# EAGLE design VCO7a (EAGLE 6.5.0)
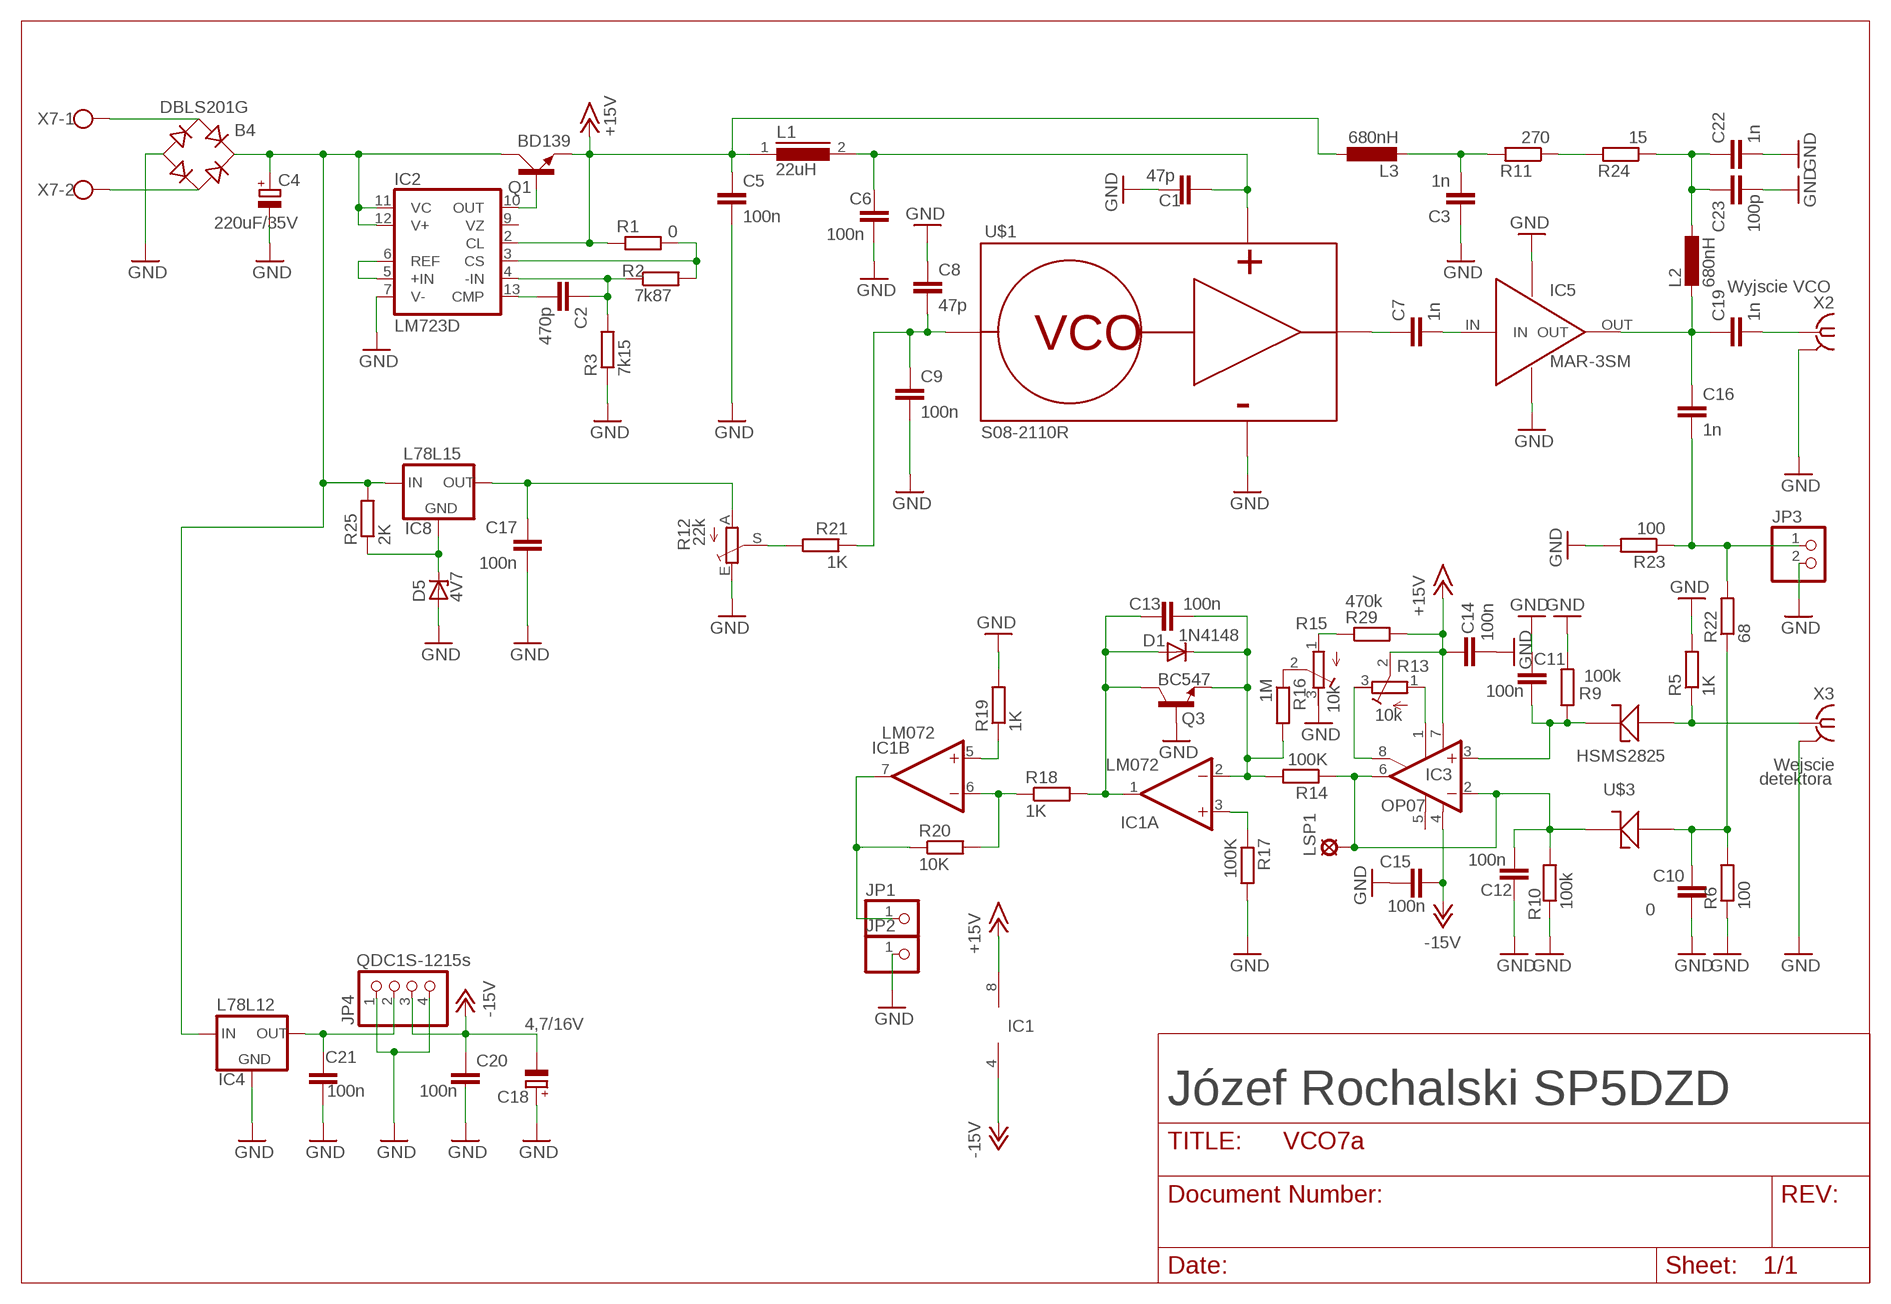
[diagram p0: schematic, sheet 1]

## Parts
B4  DBLS201G  [DBS]
C1  47p  C-EUC1812  [C1812]
C2  470p  C-EUC1206K  [C1206K]
C3  1n  C-EUC1206K  [C1206K]
C4  220uF/35V  CPOL-EU140CLH-1010  [140CLH-1010]
C5  100n  C-EUC1206K  [C1206K]
C6  100n  C-EUC1206K  [C1206K]
C7  1n  C-EUC1206K  [C1206K]
C8  47p  C-EUC1812  [C1812]
C9  100n  C-EUC1206K  [C1206K]
C10  0  C-EUC1206K  [C1206K]
C11  100n  C-EUC1206K  [C1206K]
C12  100n  C-EUC1206K  [C1206K]
C13  100n  C-EUC1206K  [C1206K]
C14  100n  C-EUC1206K  [C1206K]
C15  100n  C-EUC1206K  [C1206K]
C16  1n  C-EUC1206K  [C1206K]
C17  100n  C-EUC1206K  [C1206K]
C18  4,7/16V  CPOL-EUCT6032  [CT6032]
C19  1n  C-EUC1206  [C1206]
C20  100n  C-EUC1206K  [C1206K]
C21  100n  C-EUC1206K  [C1206K]
C22  1n  C-EUC1206K  [C1206K]
C23  100p  C-EUC1206K  [C1206K]
D1  1N4148  DIODE-MELF-MLL41  [MELF-MLL41]
D5  4V7  1N4728  [DO41Z10]
IC1  LM072  TL072D  [SO08]
IC2  LM723D  [SO14]
IC3  OP07  OP07CR  [SO08]
IC4  L78L12  L78LXXCZ/BZ  [TO92]
IC5  MAR-3SM  MMIC  [MMIC]
IC8  L78L15  L78LXXCZ/BZ  [TO92]
JP1  PINHD-1X01_2.54  [1X01]
JP2  PINHD-1X01_2.54  [1X01]
JP3  PINHD-1X2  [1X02]
JP4  QDC1S-1215s  PINHD-1X4  [1X04]
L1  22uH  EMC9714  [EMC9714]
L2  680nH  L-EUL4035M  [L4035M]
L3  680nH  L-EUL4035M  [L4035M]
LSP1  SE11  [SE11]
Q1  BD139  [TO126AV]
Q3  BC547  BC847CSMD  [SOT23]
R1  0  R-EU_R1206  [R1206]
R2  7k87  R-EU_R1206  [R1206]
R3  7k15  R-EU_R1206  [R1206]
R5  1K  R-EU_R1206  [R1206]
R6  100  R-EU_R1206  [R1206]
R9  100k  R-EU_R1206  [R1206]
R10  100k  R-EU_R1206  [R1206]
R11  270  R-EU_R1206  [R1206]
R12  22k  TRIM_EU-PT10S  [PT-10S]
R13  10k  R-TRIMM64W  [RTRIM64W]
R14  100K  R-EU_R1206  [R1206]
R15  10k  R-TRIMM64W  [RTRIM64W]
R16  1M  R-EU_R1206  [R1206]
R17  100K  R-EU_R1206  [R1206]
R18  1K  R-EU_R1206  [R1206]
R19  1K  R-EU_R1206  [R1206]
R20  10K  R-EU_R1206  [R1206]
R21  1K  R-EU_R1206  [R1206]
R22  68  R-EU_R1206  [R1206]
R23  100  R-EU_R1206  [R1206]
R24  15  R-EU_R1206  [R1206]
R25  2K  R-EU_R1206  [R1206]
R29  470k  R-EU_R1206  [R1206]
U$1  S08-2110R  [S08-2110R]
U$3  HSMS2825  [HSMS2825]
X2  SMA-142-0701-801/806  [J502-ND-142-0701-801/806]
X3  BNC  SMA-142-0701-801/806  [J502-ND-142-0701-801/806]
X7  AK300/2  [AK300/2]

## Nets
+15V: C5.1 C14.1 IC1.8(P:V+) IC2.2(CL) IC3.7(V+) L1.1 L3.1 Q1.E R1.1 R13.2(S) R29.2
-12V: C15.2 C18.- C20.1 IC1.4(P:V-) IC3.4(V-) JP4.3 ; supply symbol labelled -15V
GND: B4.- C1.2 C3.1 C4.- C5.2 C6.2 C8.1 C9.2 C10.2 C11.1 C12.2 C14.2 C15.1 C17.2 C18.+ C20.2 C21.2 C22.2 C23.2 D5.A IC2.7(V-) IC4.2(GND) IC5.GND IC5.GND1 JP2.1 JP3.2 JP4.1 JP4.4 Q3.1(B) R3.1 R5.2 R6.1 R9.2 R10.1 R12.E R15.3(E) R17.2 R19.2 R23.2 U$1.P$4(GND) X2.G@1 X2.G@2 X2.G@3 X2.G@4 X3.G@1 X3.G@2 X3.G@3 X3.G@4
N$1: IC2.5(+IN) IC2.6(REF)
N$2: IC2.10(OUT) Q1.B
N$3: R12.S R21.2
N$4: C7.1 U$1.P$3(OUT)
N$5: C2.2 IC2.13(CMP)
N$6: C2.1 IC2.4(-IN) R2.1 R3.2
N$7: IC2.3(CS) R1.2 R2.2
N$8: C16.2 JP3.1 R22.2 R23.1
N$10: C3.2 L3.2 R11.2
N$11: C17.1 IC8.1(OUT) R12.A
N$12: D5.C IC8.2(GND) R25.1
N$13: C1.1 C6.1 L1.2 U$1.P$2(VCC)
N$14: R5.1 U$3.P$4(A2) X3.1
N$15: B4.+ C4.+ IC2.11(VC) IC2.12(V+) IC4.3(IN) IC8.3(IN) Q1.C R25.2
N$17: C8.2 C9.1 R21.1 U$1.P$1(CONTROL)
N$18: C10.1 R6.2 R22.1 U$3.P$3(A1)
N$19: IC3.8(ON2) R13.3(E)
N$20: C12.1 IC3.2(-IN) IC3.6(OUT) LSP1.MP R10.2 R14.1 U$3.P$2(K1)
N$21: C13.2 D1.C IC1.2(A:-IN) Q3.2(E) R14.2 R16.2
N$22: R15.2(S) R16.1
N$23: C16.1 C19.1 IC5.OUT L2.2
N$26: IC1.3(A:+IN) R17.1
N$27: C13.1 D1.A IC1.1(A:OUT) Q3.3(C) R18.2
N$28: R11.1 R24.2
N$29: IC1.6(B:-IN) R18.1 R20.2
N$30: IC1.5(B:+IN) R19.1
N$31: IC1.7(B:OUT) JP1.1 R20.1
N$32: IC3.1(ON1) R13.1(A)
N$33: R15.1(A) R29.1
N$34: C19.2 X2.1
N$35: C22.1 C23.1 L2.1 R24.1
N$36: C21.1 IC4.1(OUT) JP4.2
N$37: C11.2 IC3.3(+IN) R9.1 U$3.P$1(K2)
N$41: C7.2 IC5.IN
N$44: B4.AC1 X7.1
N$45: B4.AC2 X7.2
Unconnected: IC2.9(VZ) IC3.5(OPT)

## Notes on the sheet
- Wyjscie VCO
- Wejscie
- detektora
- IC1
- Józef Rochalski SP5DZD

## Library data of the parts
B4 = rectifier:DB?*G: Single Phase 1.0 AMP Glass Passivated Bridge Rectifier Taiwan Semiconductor Co.,Ltd. - TSC Source: http://www.taiwansemi.com/TSCbig5/ezcatfiles/cust/img/img/db101g.pdf http://www.ts.com.tw/db/pictures/modules/PDT/PDT060207001/DBLS201G.pdf
C1-C3 C5-C17 C19-C23 = rcl:C-EU: CAPACITOR, European symbol
C4 C18 = rcl:CPOL-EU: POLARIZED CAPACITOR, European symbol
D1 = diode-1:DIODE-: DIODE
D5 = diode-1:1N4728: Z DIODE
IC1 = linear:TL072: OP AMP
IC2 = linear:*723: Positive VOLTAGE REGULATOR
IC3 = linear3:OP07*: OP AMP
IC4 IC8 = v-reg-3:L78LXXCZ/BZ: VOLTAGE REGULATOR
IC5 = MMIC1:MMIC
JP1 JP2 = pinhead-2:PINHD-1X01: PIN HEADER
JP3 = pinhead:PINHD-1X2: PIN HEADER
JP4 = pinhead:PINHD-1X4: PIN HEADER
L1 = inductors:EMC9714: INDUCTOR
L2 L3 = rcl:L-EU: INDUCTOR, European symbol
LSP1 = solpad:SE11: SOLDER PAD
Q1 = transistor-power:BD139: NPN TRANSISTOR
Q3 = transistor-npn:BC847*: NPN Transistor
R1-R3 R5 R6 R9-R11 R14 R16-R25 R29 = rcl:R-EU_: RESISTOR, European symbol
R12 = pot:TRIM_EU-: POTENTIOMETER
R13 R15 = rcl:R-TRIMM: Trimm resistor
U$1 = S08-2110R:S08-2110R: VCO AGILENT S08-2110R 0.8-1.2GHz
U$3 = HSMS2825:HSMS2825
X2 X3 = con-coax:SMA-: SMA 50 Ohm End Launch Jack Receptacle - Round Contact; MF: JOHNSON COMPONENTS; MPN: 142-0701-801; OC_FARNELL: 1608592; OC_NEWARK: 90F2624
X7 = con-ptr500+:AK300/2: CONNECTOR

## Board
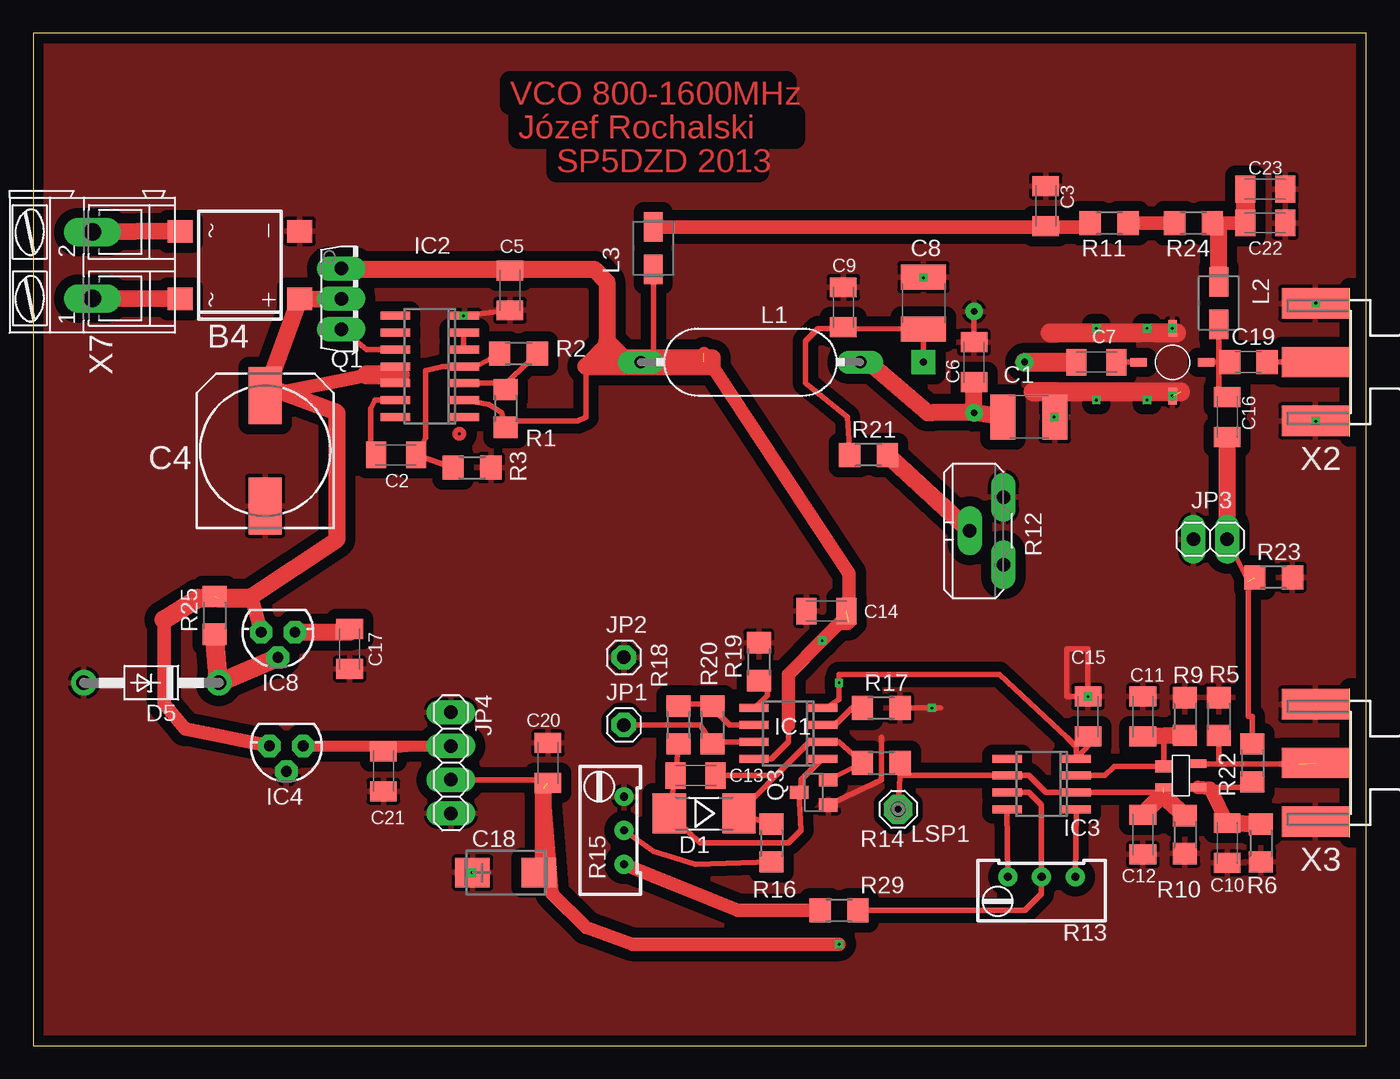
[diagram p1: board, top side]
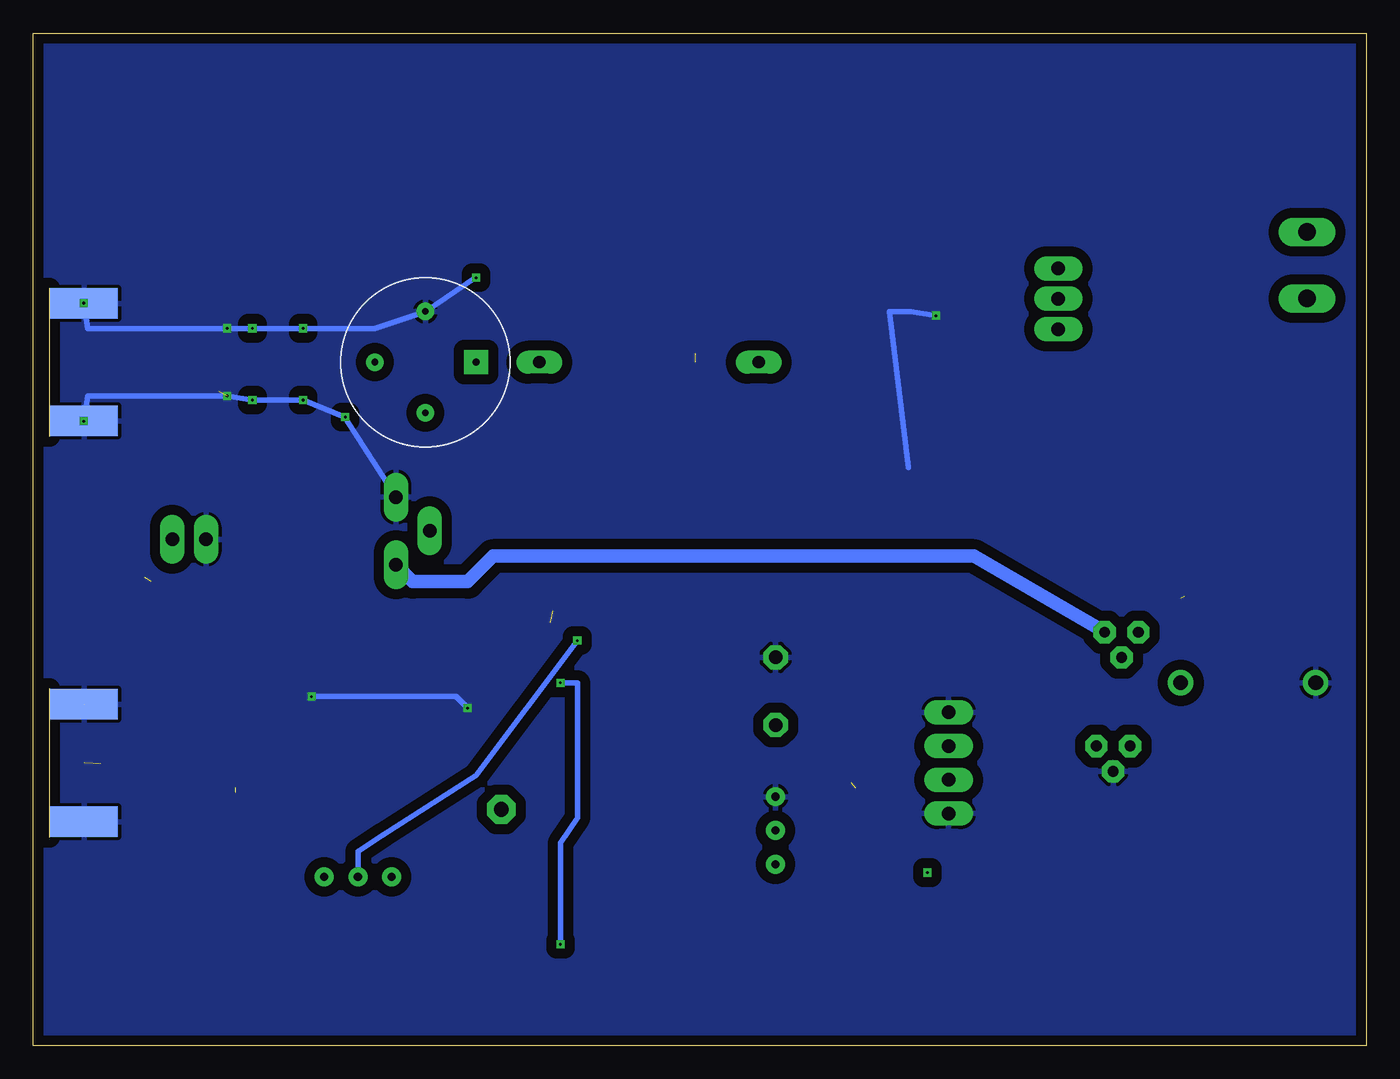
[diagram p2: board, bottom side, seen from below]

Size 100.32 x 76.19 mm. Coordinates in mm from the lower left corner, seen from the top.
Outline: 0,0 100.32,0 100.32,76.19 0,76.19 0,0
Copper layers (1*16): Top 0.035mm / dielectric 1.5mm / Bottom 0.035mm
Design rules "default *": minimum track width 16mil, minimum drill 8mil, track to track 16mil, track to pad 8mil, pad to pad 8mil, via to via 8mil, smd to smd 8mil, copper to edge 10mil, drill to drill 8mil, minimum pad ring 16mil, minimum via ring 8mil, stop-mask expansion 4mil, vias tented up to drill 0mil, thermal gap 10mil

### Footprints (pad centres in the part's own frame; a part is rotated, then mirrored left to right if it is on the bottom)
DBS = smd 1.7 x 1.9: + -2.55,-4.5; - 2.55,-4.5; AC1 -2.55,4.5; AC2 2.55,4.5
C1812 = smd 1.9 x 3.4: 1 -1.95,0; 2 1.95,0
C1206K = smd 1.5 x 2: 1 -1.5,0; 2 1.5,0
140CLH-1010 = smd 4.3 x 2.5: + 4.15,0; - -4.15,0
CT6032 = smd 2.6 x 2.2: + -2.5,0; - 2.5,0
C1206 = smd 1.6 x 1.8: 1 -1.4,0; 2 1.4,0
MELF-MLL41 = smd 2.5 x 3: A 2.625,0; C -2.625,0
DO41Z10 = drill 1.118: A 5.08,0; C -5.08,0
SO08 = smd 0.6 x 2.2: 1 -1.905,-2.6; 2 -0.635,-2.6; 3 0.635,-2.6; 4 1.905,-2.6; 5 1.905,2.6; 6 0.635,2.6; 7 -0.635,2.6; 8 -1.905,2.6
SO14 = smd 0.6 x 2.2: 1 -3.81,-2.6; 2 -2.54,-2.6; 3 -1.27,-2.6; 4 0,-2.6; 5 1.27,-2.6; 6 2.54,-2.6; 7 3.81,-2.6; 8 3.81,2.6; 9 2.54,2.6; 10 1.27,2.6; 11 0,2.6; 12 -1.27,2.6; 13 -2.54,2.6; 14 -3.81,2.6
TO92 = drill 0.813 pad 1.676 octagon: 1 -1.27,0; 2 0,1.905; 3 1.27,0
MMIC = smd 0.635 x 1.27: GND 0,2.54; GND1 0,-2.54 | smd 1.27 x 0.635: IN -2.54,0; OUT 2.54,0
1X01 = drill 1.016 octagon: 1 0,0
1X02 = drill 1.016 long: 1 -1.27,0; 2 1.27,0
1X04 = drill 1.016 long: 1 -3.81,0; 2 -1.27,0; 3 1.27,0; 4 3.81,0
EMC9714 = drill 0.914 long: 1 -8.255,0; 2 8.255,0
L4035M = smd 2.2 x 1.4: 1 -1.6,0; 2 1.6,0
SE11 = drill 1.118 pad 2.159 octagon: MP 0,0
TO126AV = drill 1.016 long: B 2.286,-1.27; C 0,-1.27; E -2.286,-1.27
SOT23 = smd 1 x 1.4: 1 -0.95,-1.1; 2 0.95,-1.1; 3 0,1.1
R1206 = smd 1.6 x 1.803: 1 -1.422,0; 2 1.422,0
PT-10S = drill 1.016 long: A -2.54,-1.27; E 2.54,-1.27; S 0,1.27
RTRIM64W = drill 0.61: 1 1.27,-2.54; 2 1.27,0; 3 1.27,2.54
S08-2110R = drill 0.5 pad 1.778 square: P$1 -3.81,0 | drill 0.5 pad 1.27: P$2 0,3.81; P$3 3.81,0; P$4 0,-3.81
HSMS2825 = smd 0.914 x 1.27: P$1 -0.699,-1.27 | smd 0.635 x 1.27: P$2 0.889,-1.27; P$3 0.889,1.27; P$4 -0.889,1.27
J502-ND-142-0701-801/806 = smd 5.08 x 2.286: 1 2.565,0; G@1 2.565,4.42; G@2 2.565,-4.42 | smd 5.08 x 2.286 bottom: G@3 2.565,4.42; G@4 2.565,-4.42
AK300/2 = drill 1.321 long: 1 -2.515,0; 2 2.489,0

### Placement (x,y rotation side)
B4  15.56,58.74 90 top
C1  74.93,47.31 0 top
C2  27.3,44.45 180 top
C3  76.2,63.18 270 top
C4  17.46,44.77 90 top
C5  35.88,56.83 270 top
C6  70.8,51.44 90 top
C7  80.01,51.44 0 top
C8  66.99,55.88 270 top
C9  60.96,55.56 90 top
C10  89.85,15.24 270 top
C11  83.5,24.77 270 top
C12  83.5,15.88 270 top
C13  49.85,20.32 0 top
C14  59.69,32.7 180 top
C15  79.38,24.77 270 top
C16  89.85,47.31 270 top
C17  23.81,29.84 270 top
C18  35.56,13.02 0 top
C19  91.44,51.44 0 top
C20  38.73,21.27 90 top
C21  26.35,20.64 270 top
C22  92.71,61.91 0 top
C23  92.71,64.45 0 top
D1  50.48,17.46 180 top
D5  8.89,27.3 180 top
IC1  56.83,23.5 90 top
IC2  29.84,51.12 90 top
IC3  75.88,19.68 90 top
IC4  19.05,22.54 180 top
IC5  85.72,51.44 0 top
IC8  18.41,31.11 180 top
JP1  44.45,24.13 0 top
JP2  44.45,29.21 0 top
JP3  88.58,38.1 180 top
JP4  31.43,21.27 270 top
L1  53.98,51.44 0 top
L2  89.22,55.88 270 top
L3  46.67,60.01 90 top
LSP1  65.09,17.78 0 top
Q1  24.45,56.2 270 top
Q3  58.74,19.05 90 top
R1  35.56,47.94 90 top
R2  36.51,52.07 0 top
R3  33.02,43.5 180 top
R5  89.22,24.77 90 top
R6  92.39,15.24 90 top
R9  86.68,24.77 90 top
R10  86.68,15.88 90 top
R11  80.96,61.91 180 top
R12  71.75,38.73 90 top
R13  75.88,11.43 90 top
R14  63.82,21.27 180 top
R15  43.18,16.19 0 top
R16  55.56,15.24 90 top
R17  63.82,25.4 0 top
R18  48.58,24.13 270 top
R19  54.61,28.89 90 top
R20  51.12,24.13 90 top
R21  62.87,44.45 0 top
R22  91.76,21.27 90 top
R23  93.34,35.24 0 top
R24  87.31,61.91 180 top
R25  13.65,32.38 90 top
R29  60.64,10.16 0 top
U$1  70.8,51.44 180 bottom
U$3  86.36,20.32 270 top
X2  99.06,51.44 180 top
X3  99.06,21.27 180 top
X7  4.45,58.74 90 top

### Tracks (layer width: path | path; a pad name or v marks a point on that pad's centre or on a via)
+15V  (via drill 0.2)  (2 unrouted)
  Top 0.406: IC2.2 34.29,48.26 35.24,47.62 R1.1 36.03,46.99 40.96,46.99 41.59,47.31 41.59,51.12 43.18,51.12 | 51.43,51.12 51.12,51.12 50.8,51.12 | 50.8,51.12 46.67,51.12 | 46.67,51.12 43.18,51.12 | 41.91,58.42 35.97,58.42 C5.1 35.73,58.48 Q1.E | 50.8,51.12 L1.1 | 43.18,53.02 43.18,51.12 | L3.1 46.67,51.12 | IC1.8 55.56,21.59 56.83,22.86 56.83,24.13 | IC3.7 74.93,19.05 75.88,18.1 R13.2 75.88,11.43 74.61,10.16 R29.2
  Top 1.016: 50.48,52.07 61.39,35.54 61.39,31.86 61.28,31.75 60.64,31.75 v59.37,30.48 56.83,27.94 56.83,24.13
  Top 1.27: 23.18,58.42 41.91,58.42 42.23,58.42 43.18,57.47 43.18,53.02 | 43.18,53.02 43.18,52.7 41.59,51.12 46.67,51.12 51.12,51.12 51.12,51.44 | 51.12,51.44 51.12,51.75 44.45,51.75 | 43.5,51.75 44.45,51.75 | 44.45,51.75 43.18,53.02 | 50.48,51.44 51.12,51.44
  Bottom 0.406: v59.37,30.48 66.99,20.32 73.98,15.88 75.88,14.61 R13.2
-12V  (via drill 0.2)  (1 unrouted)
  Top 0.406: JP4.3 38.73,20 C20.1 | C15.2 79.46,23.18 80.01,23.18 78.48,21.65 IC3.4 78.48,22.48 77.79,23.18 72.71,27.94 60.64,27.94 v60.64,27.3 60.64,26.04 59.69,25.4 IC1.4 59.37,25.4
  Top 1.016: 38.42,19.37 39.05,11.43 41.59,8.89 45.08,7.62 v60.64,7.62
  Top 1.27: C18.- 38.42,13.02 38.42,19.37
  Bottom 0.406: v60.64,7.62 60.64,15.24 59.37,17.14 59.37,27.3 v60.64,27.3
GND  (via drill 0.2)  (2 unrouted)
  Top 0.406: U$1.P$4 C6.2 | C5.2 IC2.7 v32.39,54.93 | Q3.1 63.82,20 63.82,23.18 | C15.1 79.38,26.04 | C15.1 79.38,26.35 79.06,26.04 | R19.2 54.76,30.31 54.93,30.48 54.29,30.48 | 65.09,25.4 R17.2 v67.63,25.4 68.26,25.4 | C15.1 77.79,26.27 77.79,29.84 79.38,29.84 C15.1
  Top 1.422: 76.52,53.66 86.04,53.66 | 75.25,49.21 86.36,49.21
  Bottom 0.406: JP4.4 31.43,17.14 | v67.63,25.4 68.49,26.27 C15.1 | v32.39,54.93 34.29,55.24 35.88,55.24 R3.1 | R12.E C1.2 80.01,48.58 83.82,48.58 IC5.GND1 96.2,48.9 X2.G@3 | C8.1 U$1.P$4 74.61,53.98 IC5.GND 96.2,53.98 X2.G@4
  other vias: 85.72,53.98 79.38,26.27 85.72,48.9
  pour Top (isolate 0.762): 0.32,76.2 100.65,76.2 100.65,0 0.32,0
  pour Bottom (isolate 0.762): -1.59,78.11 101.92,78.11 101.92,-1.91 -1.59,-1.91
N$1
  Top 0.406: IC2.5 32.39,52.39 32.39,53.66 IC2.6
N$2
  Top 0.406: Q1.B 25.08,52.39 IC2.10
N$3
  Top 1.27: R12.S R21.2
N$4
  Top 1.422: U$1.P$3 C7.1
N$5
  Top 0.406: IC2.13 25.72,48.58 25.4,47.94 25.4,44.77 C2.2
N$6
  Top 0.406: R2.1 33.34,51.12 IC2.4 30.8,51.12 29.53,50.8 29.53,45.72 C2.1 R3.2
N$7
  Top 0.406: IC2.3 34.93,49.85 35.52,49.78 | 35.52,49.78 R2.2 | R1.2 35.56,49.53 35.52,49.78
N$8  (1 unrouted)
  Top 0.406: JP3.1 91.44,34.92 91.44,24.77 91.76,24.77 R22.2
  Top 1.27: JP3.1 C16.2
N$9
  Top 1.422: 25.08,50.48 27.62,50.48
N$10
  Top 0.406: 79.24,61.61 79.25,61.59 79.38,61.59 | C3.2 76.43,61.91 R11.2
  Top 1.016: L3.2 46.67,62.23 | L3.2 46.67,61.91 | R11.2 79.24,61.61 L3.2
N$11
  Top 1.27: IC8.1 23.81,31.11 C17.1
  Bottom 1.016: IC8.1 29.53,36.83 65.72,36.83 67.63,34.92 71.76,34.92 R12.A
N$12
  Top 0.406: D5.C R25.1
  Top 1.422: IC8.2 D5.C 13.65,30.8
N$13
  Top 0.406: U$1.P$2 C1.1 | 70.8,49.85 C6.1 | L1.2 62.86,51.44 67.63,47.62
  Top 1.27: 73.02,47.31 U$1.P$2 | U$1.P$2 67.63,47.62 | U$1.P$2 70.8,49.85
N$14  (1 unrouted)
  Top 0.406: U$3.P$4 89.22,21.21 | 89.22,21.21 95.25,21.21 95.25,21.27 | R5.1 89.22,21.21
N$15  (1 unrouted)
  Top 0.406: IC2.12 27.31,49.85 27.31,50.48 27.31,51.12 IC2.11
  Top 1.016: C4.+ 25.4,50.48 27.31,50.48 | IC4.3 11.43,23.81 9.84,25.72 9.84,32.07 | IC8.3 16.41,33.8
  Top 1.27: C4.+ 17.64,49.57 | 17.64,49.57 B4.+ Q1.C | 16.19,33.66 16.41,33.8 22.86,38.1 22.86,47.62 17.64,49.57
  Top 1.422: 16.19,33.66 13.97,33.66 | 9.84,32.07 12.38,33.66 R25.2
N$16
  Top 1.27: 67.31,47.62 62.86,51.44
N$17
  Top 0.406: U$1.P$1 C8.2 61.6,53.98 | R21.1 61.28,47.31 58.1,49.85 58.1,53.02 59.05,53.98 61.6,53.98 | 61.6,53.98 C9.1
N$18
  Top 0.406: U$3.P$3 91.76,19.43 R22.1
  Top 1.016: C10.1 88.7,19.12 88.58,19.37 U$3.P$3
  Top 1.27: R6.2 C10.1
N$19
  Top 0.406: IC3.8 R13.3
N$20  (1 unrouted)
  Top 0.406: LSP1.MP 65.17,19.39 65.21,20.34 | 65.21,20.34 R14.1 | 65.21,20.34 65.22,20.32 IC3.6 74.93,20.32 76.2,19.05 IC3.2 84.47,19.05 84.79,18.73
  Top 1.27: 85.09,19.05 84.92,18.87 | 84.92,18.87 84.79,18.73 C12.1 | R10.2 84.92,18.87
N$21
  Top 0.406: 55.88,20.32 C13.2 | 55.88,20.32 58.42,22.86 IC1.2 60.64,22.86 R14.2 Q3.2 | 55.88,20.32 D1.C R16.2
N$22
  Top 0.406: R15.2 46.67,14.61 49.85,13.65 R16.1
N$23
  Top 0.406: IC5.OUT 89.22,51.44 | L2.2 89.22,51.44 | 89.22,51.44 89.22,48.9 C16.1 | C19.1 89.22,51.44
N$26
  Top 0.406: R17.1 61.6,25.4 60.33,24.13 IC1.3
N$27
  Top 0.406: IC1.1 59.37,21.59 57.79,20 57.79,19.05 Q3.3 57.79,16.19 56.83,15.24 50.16,15.24 D1.A C13.1 R18.2
N$28
  Top 1.016: R11.1 R24.2
N$29
  Top 0.406: R18.1 48.58,25.72 51.12,25.72 R20.2 51.12,25.4 52.39,24.13 IC1.6
N$30
  Top 0.406: R19.1 55.25,27.94 55.25,26.35 54.29,25.4 IC1.5
N$31
  Top 0.406: IC1.7 51.12,22.86 R20.1 50.16,24.13 JP1.1
N$32
  Top 0.406: IC3.1 R13.1
N$33
  Top 1.016: R15.1 53.02,10.16 R29.1
N$34
  Top 0.406: C19.2 X2.1
N$35
  Top 1.016: C22.1 R24.1
  Top 1.27: L2.1 89.22,61.59 88.9,61.91 R24.1
  Top 1.422: C23.1 C22.1
N$36
  Top 0.406: 26.35,21.59 C21.1 JP4.2
  Top 0.813: IC4.1 JP4.2
N$37
  Top 0.406: IC3.3 80.65,20.32 81.34,21.02 U$3.P$1 85.09,23.29 85.08,23.3
  Top 1.27: R9.1 85.08,23.3 C11.2
N$38  (via drill 0.2)
  other vias: 76.83,47.31
N$39  (via drill 0.2)
  other vias: 96.52,55.88
N$40  (via drill 0.2)
  other vias: 96.52,46.99
N$41
  Top 0.406: C7.2 IC5.IN
N$42  (via drill 0.2)
  other vias: 66.99,57.78
N$44
  Top 1.27: B4.AC1 X7.1
N$45
  Top 1.27: B4.AC2 X7.2
N$47  (via drill 0.2)
  other vias: 80.01,53.98
N$49  (via drill 0.2)
  other vias: 83.82,53.98
N$53  (via drill 0.2)
  other vias: 83.82,48.58
N$54  (via drill 0.2)
  other vias: 80.01,48.58
N$56  (via drill 0.2)
  other vias: 33.02,13.02
(copper drawn outside any net)
  shapes: Top circle x1

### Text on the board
Top: VCO 800-1600MHz | Józef Rochalski | SP5DZD 2013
